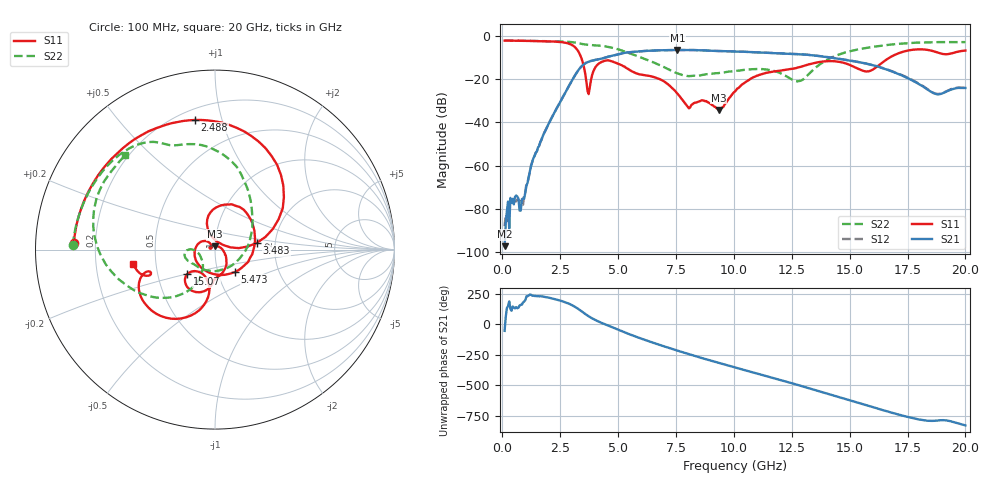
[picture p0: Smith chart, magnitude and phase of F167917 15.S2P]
!  2-Port S-parameters saved by WinCal
! VAR MeasName=S-Parameters (CALIBRATED_DATA) read from VNA (N5242A)
! VAR MeasDate=2016-11-22 9:00:24
! VAR NAME=F167917 15
! VAR FILENAME=F167917 15.S2P
! VAR DATE=2016-11-22 9:00:24
! VAR PHYS_PORTS=1,2
# Hz S DB R 50
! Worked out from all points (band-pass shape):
!   401 points, 100 MHz to 20 GHz, reference 50 ohm
!   highest |S21| = -6.44 dB at 7.562 GHz (marker M1); lowest = -97.4 dB at 100 MHz (marker M2)
!   |S21| within 3 dB of the highest: 4.616 GHz to 13.81 GHz (9.193 GHz wide, 99.8 % of centre)
!   lowest |S11| = -34.3 dB at 9.354 GHz (marker M3), VSWR 1.04, Z = 49.9 + j1.93 ohm
!   |S11| at or under -10 dB: 3.408 GHz to 16.72 GHz (13.32 GHz wide, 132 % of centre)
!   |S22| runs from -21.0 to -2.0 dB; largest |S21 - S12| = 0.0045
!   S11 on the Smith chart (normalised r, x): 100 MHz: 0.12, +0.02; 2.488 GHz: 0.27, +0.82; 3.483 GHz: 1.61, +0.13; 5.473 GHz: 1.21, -0.31; 15.07 GHz: 0.71, -0.20; 20 GHz: 0.37, -0.07
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1e8  -2.08 177.3  -97.40 -54.6  -88.15 60.0  -2.03 178.3
8.4625e8  -2.19 157.4  -75.59 159.6  -77.91 128.4  -2.13 166.4
1.34375e9  -2.28 143.3  -56.58 -126.3  -56.81 -124.9  -2.21 158.4
2.488e9  -2.72 98.7  -30.80 -166.2  -30.81 -166.7  -2.45 137.7
3.43325e9  -10.73 14.2  -13.92 104.0  -13.92 104.0  -3.63 116.2
3.483e9  -12.49 9.2  -13.44 97.2  -13.42 97.1  -3.73 115.4
3.73175e9  -26.90 72.3  -11.88 64.6  -11.86 64.5  -4.08 111.8
4.32875e9  -11.82 77.7  -10.34 7.6  -10.33 7.3  -4.58 98.3
5.473e9  -15.51 -47.8  -7.50 -80.8  -7.49 -81.0  -7.87 65.0
6.7665e9  -19.81 165.2  -6.58 -167.8  -6.59 -167.9  -13.34 21.5
7.5625e9  -26.64 128.3  -6.44 143.8  -6.47 143.7  -17.28 -30.8
8.01025e9  -32.81 143.2  -6.48 117.9  -6.48 117.9  -18.52 -70.7
9.3535e9  -34.27 91.1  -6.92 43.3  -6.93 43.3  -17.12 -141.2
1.005e10  -25.67 -15.8  -7.12 6.0  -7.14 6.1  -16.24 -153.8
1.17415e10  -16.38 -83.8  -7.90 -82.8  -7.86 -82.6  -16.15 -178.6
1.27365e10  -14.63 -93.6  -8.35 -136.2  -8.33 -136.1  -20.99 -154.9
1.338325e10  -12.71 -102.2  -8.90 -172.5  -8.85 -172.3  -16.08 -118.8
1.507475e10  -13.71 -138.4  -11.46 94.1  -11.43 94.0  -6.88 -145.4
1.5821e10  -16.34 -116.1  -13.00 51.3  -13.00 51.9  -5.31 -159.8
1.67165e10  -10.05 -101.3  -15.89 1.1  -15.82 1.6  -4.00 -175.9
1.87065e10  -7.29 -160.4  -26.79 -70.4  -26.66 -70.8  -2.80 150.5
2e10  -6.71 -170.3  -24.06 -109.1  -23.92 -109.7  -2.79 133.5
